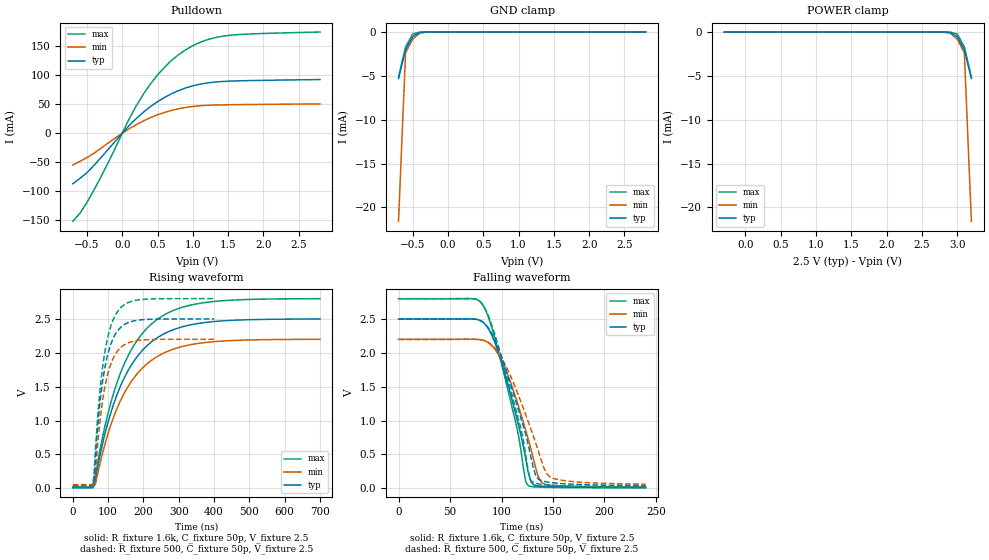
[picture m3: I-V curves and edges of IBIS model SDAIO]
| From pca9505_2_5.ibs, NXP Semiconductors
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[Model]   SDAIO
Model_type I/O_open_drain
Vinh=1.5
Vinl=0.75
Vref=2.5
Vmeas=1.25
Rref=1.6k
Cref=50p
C_comp   7p   6.8p   7.2p
[Temperature Range] 27   85   -40
[Voltage Range]   2.5   2.2   2.8
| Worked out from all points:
|   slope of the pulldown table from 0 to 0.375 V, typ, clamps not added: 8.64 ohm
|   GND clamp passes 1 mA (typ) near -0.53 V on its own axis
|   falling waveform, R_fixture 1.6k, C_fixture 50p, V_fixture 2.5: 20-80 % time 25.5ns typ, 26.9ns min, 25.7ns max; typ from 2.5 V to 0.013 V
|   falling waveform, R_fixture 500, C_fixture 50p, V_fixture 2.5: 20-80 % time 29.2ns typ, 31.7ns min, 28.6ns max; typ from 2.5 V to 0.04 V
|   rising waveform, R_fixture 1.6k, C_fixture 50p, V_fixture 2.5: 20-80 % time 113ns typ, 114ns min, 113ns max; typ from 0.011 V to 2.5 V
|   rising waveform, R_fixture 500, C_fixture 50p, V_fixture 2.5: 20-80 % time 35.5ns typ, 35.6ns min, 35.4ns max; typ from 0.036 V to 2.5 V
[Pulldown]
-700mV    -86.88mA   -54.63mA   -151.4mA
-600mV    -77.73mA   -48.46mA   -137.8mA
-400mV    -55.28mA   -34.48mA   -97.51mA
-200mV    -27.91mA   -16.94mA   -50.79mA
100mV     13.33mA    7.793mA    25mA
300mV     36.19mA    21.16mA    67.22mA
500mV     54.27mA    31.61mA    100.2mA
800mV     73.4mA     42.13mA    135.2mA
1.1V      84.29mA    47.18mA    156.2mA
1.4V      88.79mA    48.71mA    166.4mA
1.8V      90.48mA    49.38mA    170.6mA
2.8V      92.24mA    50.35mA    173.9mA
[GND Clamp]
-700mV    -5.302mA   -21.58mA   -5.122mA
-600mV    -2.04mA    -2.358mA   -1.687mA
-500mV    -525.2uA   -816.9uA   -228.9uA
-400mV    -48.21uA   -135uA     -7.763uA
-200mV    -27.28nA   -200nA     -811.9pA
2.8V      51pA       210.6pA    36.58pA
[POWER Clamp]
-300mV    51pA       210.6pA    36.58pA
2.7V      -27.28nA   -200nA     -811.9pA
2.9V      -48.21uA   -135uA     -7.763uA
3V        -525.2uA   -816.9uA   -228.9uA
3.1V      -2.04mA    -2.358mA   -1.687mA
3.2V      -5.302mA   -21.58mA   -5.122mA
[Falling Waveform]
R_fixture=1.6k
C_fixture=50p
V_fixture=2.5
V_fixture_min=2.2
V_fixture_max=2.8
0s        2.5V       2.2V       2.8V
82.42ns   2.448V     2.185V     2.692V
92.12ns   2.207V     2.084V     2.294V
101.8ns   1.773V     1.833V     1.73V
116.4ns   944mV      1.219V     796.3mV
123.6ns   423.9mV    850.6mV    93.62mV
126.1ns   228.1mV    720.7mV    36.81mV
135.8ns   36.12mV    170.2mV    18.93mV
140.6ns   30.44mV    69.41mV    16.25mV
240ns     12.6mV     19.45mV    7.348mV
[Falling Waveform]
R_fixture=500
C_fixture=50p
V_fixture=2.5
V_fixture_min=2.2
V_fixture_max=2.8
0s        2.5V       2.2V       2.8V
72.73ns   2.5V       2.201V     2.8V
82.42ns   2.451V     2.186V     2.699V
101.8ns   1.862V     1.881V     1.84V
118.8ns   1.04V      1.281V     887.8mV
126.1ns   636.4mV    980.7mV    247.2mV
130.9ns   299.8mV    773.5mV    86.91mV
140.6ns   106mV      322.6mV    55.61mV
147.9ns   85.93mV    162.4mV    46.05mV
240ns     40.49mV    62.51mV    23.6mV
[Rising Waveform]
R_fixture=1.6k
C_fixture=50p
V_fixture=2.5
V_fixture_min=2.2
V_fixture_max=2.8
0s        11.23mV    16.9mV     6.677mV
56.57ns   12.58mV    17.41mV    6.506mV
63.64ns   131.8mV    53.17mV    167.7mV
98.99ns   960.2mV    794.2mV    1.091V
134.3ns   1.5V       1.285V     1.691V
176.8ns   1.904V     1.655V     2.141V
233.3ns   2.202V     1.926V     2.471V
297ns     2.363V     2.074V     2.649V
374.7ns   2.447V     2.151V     2.742V
700ns     2.499V     2.199V     2.799V
[Rising Waveform]
R_fixture=500
C_fixture=50p
V_fixture=2.5
V_fixture_min=2.2
V_fixture_max=2.8
0s        35.92mV    53.95mV    21.37mV
56.57ns   43.01mV    57.09mV    23.24mV
60.61ns   163.5mV    93.81mV    233.4mV
64.65ns   500.6mV    255.5mV    608.1mV
72.73ns   1.041V     776.5mV    1.202V
88.89ns   1.724V     1.441V     1.952V
105.1ns   2.088V     1.796V     2.35V
129.3ns   2.34V      2.043V     2.626V
189.9ns   2.485V     2.185V     2.784V
400ns     2.5V       2.2V       2.8V
[Ramp]
R_load=1.6k
dV/dt_r   1.493E+0/2.907E-9   1.488E+0/3.494E-9   1.496E+0/2.561E-9
dV/dt_f   1.493E+0/2.362E-8   1.487E+0/2.765E-8   1.496E+0/2.141E-8
|[End   SDAIO
